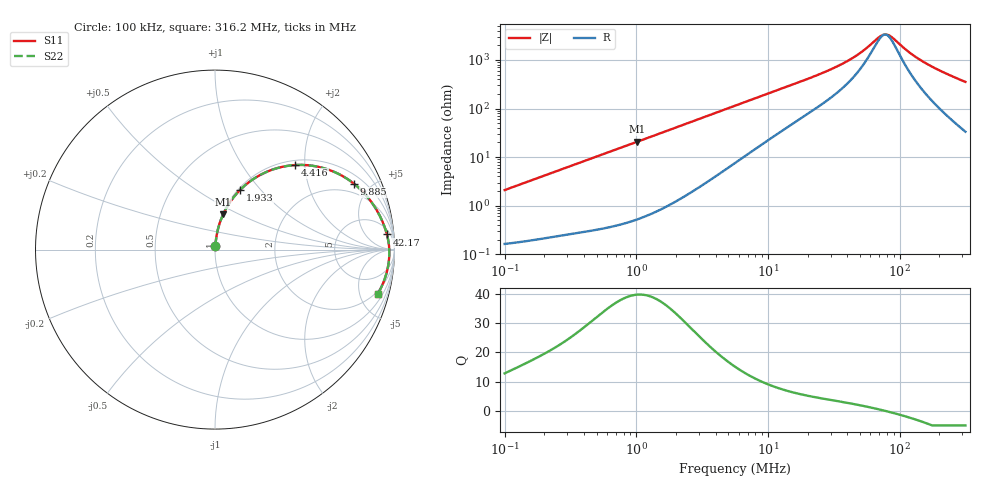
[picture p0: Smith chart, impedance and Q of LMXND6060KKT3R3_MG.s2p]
! LMXND6060KKT3R3_MG  S-PARAMETER MODEL  ( General Type )
! Model Generated by TAIYO YUDEN Corporation (https://www.yuden.co.jp/en/)
! Version 1.0
! TAIYO YUDEN Control No. 191023NI43SB-FBB
! Copyright(c) 2019 TAIYO YUDEN CO.,LTD. All Rights Reserved.
! Product Description (link to TY-COMPAS)
! https://ds.yuden.co.jp/TYCOMPAS/or/detail?pn=LMXND6060KKT3R3MMG&u=M
! Products Name : Inductors
! Characteristics :
!  Inductance : 3.3 uH , SRF(min) : 42 MHz , DC Resistance(max) : 0.162 Ohm
!  Rated Current : Saturation :1600 mA , Temp Rise : 1500 mA (40 degC)
!  Case Size : 6.0 x 6.0 / 0.236 x 0.236 [mm/inch] , Thickness : 1 / 0.039 [mm/inch]
!  (Conditions: Temperature = 25 degC , DC Bias Current/Voltage = 0A / 0V)
! External Node Assignments :
!  1  o---GGG---o  2
! GND o---------o GND
! Frequency Range : 0.1MHz  -  316.199832MHz  [ 402 STEP ]
# MHz S RI R 50
! Freq[MHz].  S11 Real  S11 Imag  S21 Real  S21 Imag  S12 Real  S12 Imag  S22 Real  S22 Imag
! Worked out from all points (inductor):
!   401 points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, 100 kHz to 316.2 MHz, reference 50 ohm
!   read as one part in series: L = 3.31 uH near 104.1 kHz
!   highest Q = 39.7 at 1.014 MHz (marker M1), where L = 3.24 uH
!   self-resonance near 77.43 MHz
!   S11 on the Smith chart (normalised r, x): 100 kHz: 1.00, +0.04; 1.933 MHz: 1.02, +0.78; 4.416 MHz: 1.10, +1.79; 9.885 MHz: 1.43, +3.97; 42.17 MHz: 8, +19; 316.2 MHz: 1.67, -7.04
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0.1  0.00206 0.0208  0.9979 -0.0208  0.9979 -0.0208  0.00206 0.0208
0.385695  0.00896 0.078  0.991 -0.078  0.991 -0.078  0.00896 0.078
0.638251  0.0201 0.127  0.9799 -0.127  0.9799 -0.127  0.0201 0.127
1.014469  0.0454 0.1959  0.9546 -0.1959  0.9546 -0.1959  0.0454 0.1959
1.487603  0.0897 0.2729  0.9103 -0.2729  0.9103 -0.2729  0.0897 0.2729
1.933018  0.1408 0.3333  0.8592 -0.3333  0.8592 -0.3333  0.1408 0.3333
2.83455  0.2566 0.4183  0.7434 -0.4183  0.7434 -0.4183  0.2566 0.4183
4.415521  0.4477 0.4711  0.5523 -0.4711  0.5523 -0.4711  0.4477 0.4711
5.623165  0.5607 0.4642  0.4393 -0.4642  0.4393 -0.4642  0.5607 0.4642
9.885033  0.7752 0.3664  0.2248 -0.3664  0.2248 -0.3664  0.7752 0.3664
14.20615  0.8585 0.2822  0.1415 -0.2822  0.1415 -0.2822  0.8585 0.2822
21.68824  0.9152 0.1938  0.0848 -0.1938  0.0848 -0.1938  0.9152 0.1938
31.80333  0.9446 0.1271  0.0554 -0.1271  0.0554 -0.1271  0.9446 0.1271
42.16686  0.9581 0.0842  0.0419 -0.0842  0.0419 -0.0842  0.9581 0.0842
52.6284  0.965 0.0527  0.035 -0.0527  0.035 -0.0527  0.965 0.0527
71.19815  0.9703 0.0114  0.0297 -0.0114  0.0297 -0.0114  0.9703 0.0114
77.17353  0.971 0.000456  0.029 -0.000456  0.029 -0.000456  0.971 0.000456
83.65039  0.9713 -0.0106  0.0287 0.0106  0.0287 0.0106  0.9713 -0.0106
117.8193  0.9691 -0.0594  0.0309 0.0594  0.0309 0.0594  0.9691 -0.0594
150.0428  0.9635 -0.0975  0.0365 0.0975  0.0365 0.0975  0.9635 -0.0975
211.3312  0.9469 -0.1597  0.0531 0.1597  0.0531 0.1597  0.9469 -0.1597
316.1998  0.9058 -0.2485  0.0942 0.2485  0.0942 0.2485  0.9058 -0.2485
